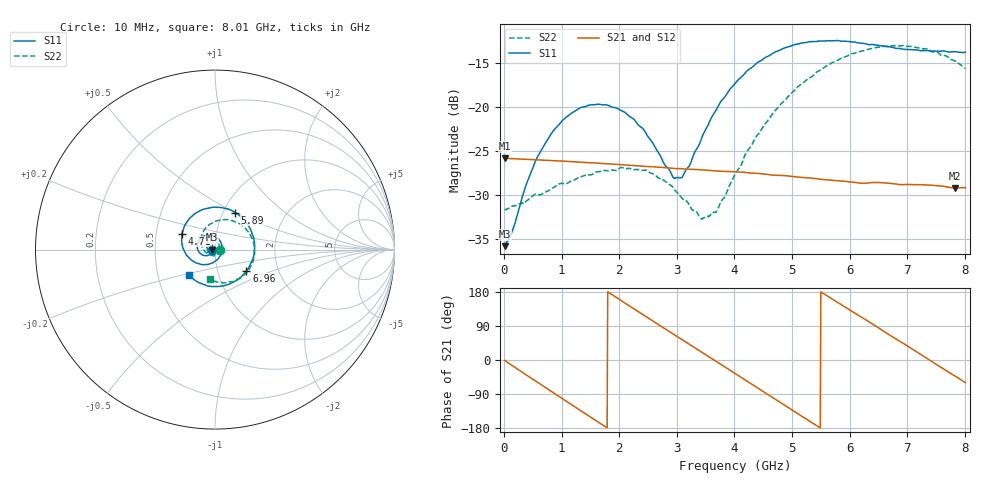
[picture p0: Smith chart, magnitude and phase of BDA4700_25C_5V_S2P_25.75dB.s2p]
!Agilent Technologies,E5071B,MY42404982,A.09.10
!Date: Mon Oct 20 13:39:27 2025
!Data & Calibration Information:
!Freq	S11:SOLT2(ON)	S21:SOLT2(ON)	S12:SOLT2(ON)	S22:SOLT2(ON)
# Hz S RI R 50
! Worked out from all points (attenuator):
!   801 points, 10 MHz to 8.01 GHz, reference 50 ohm
!   highest |S21| = -25.83 dB at 10 MHz (marker M1); lowest = -29.2 dB at 7.83 GHz (marker M2)
!   lowest |S11| = -35.8 dB at 10 MHz (marker M3), VSWR 1.03, Z = 48.4 - j0.122 ohm
!   |S11| at or under -10 dB: start of sweep to end of sweep
!   |S22| runs from -32.8 to -13.1 dB; largest |S21 - S12| = 0.00041
!   S11 on the Smith chart (normalised r, x): 10 MHz: 0.97, -0.00; 4.71 GHz: 0.68, +0.13; 5.89 GHz: 1.14, +0.50; 6.96 GHz: 1.38, -0.34; 8.01 GHz: 0.72, -0.21
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1e7  -0.0162 -0.00126  0.0511 -0.0011  0.0511 -0.00113  0.0261 -0.000799
1.4e8  -0.0173 -0.00935  0.0491 -0.0127  0.0491 -0.0127  0.0265 -0.00676
6.1e8  -0.0422 -0.0336  0.0236 -0.044  0.0236 -0.044  0.0122 -0.0293
1.01e9  -0.0799 -0.0237  -0.01 -0.0481  -0.01 -0.0482  -0.0152 -0.0335
1.35e9  -0.0989 0.0093  -0.0346 -0.0339  -0.0346 -0.034  -0.0361 -0.0178
2.08e9  -0.0466 0.0812  -0.0414 0.0218  -0.0415 0.0218  -0.0298 0.0335
2.68e9  0.0294 0.0464  -0.00284 0.0453  -0.00282 0.0453  0.0128 0.0374
2.94e9  0.0391 0.00656  0.0165 0.0416  0.0166 0.0415  0.0249 0.024
3.09e9  0.0353 -0.0183  0.0263 0.0359  0.0262 0.0359  0.0277 0.0124
3.41e9  0.00159 -0.0635  0.0405 0.017  0.0406 0.017  0.0203 -0.0115
3.54e9  -0.0196 -0.0759  0.043 0.00763  0.043 0.00757  0.0129 -0.0201
3.7e9  -0.052 -0.083  0.043 -0.00405  0.043 -0.00416  -0.000697 -0.0259
4.01e9  -0.1171 -0.0674  0.0349 -0.0248  0.0349 -0.0248  -0.0322 -0.0257
4.71e9  -0.1844 0.089  -0.00968 -0.0397  -0.00958 -0.0398  -0.0796 0.0526
5.35e9  -0.0596 0.226  -0.0381 -0.00965  -0.0381 -0.00975  -0.0153 0.1478
5.89e9  0.1129 0.206  -0.03 0.0231  -0.03 0.023  0.1047 0.1586
6.26e9  0.197 0.1147  -0.0115 0.035  -0.0111 0.0351  0.1809 0.1036
6.68e9  0.2167 -0.0298  0.0142 0.034  0.0142 0.034  0.2194 -5.25e-05
6.96e9  0.1752 -0.118  0.0273 0.0238  0.0274 0.0236  0.2082 -0.0752
7.39e9  0.0508 -0.2005  0.0359 -0.000281  0.0359 -0.000379  0.1319 -0.1625
7.83e9  -0.0989 -0.1798  0.0257 -0.0232  0.0256 -0.0234  0.0134 -0.1813
8.01e9  -0.1468 -0.1409  0.0175 -0.03  0.0176 -0.0301  -0.0302 -0.1617
